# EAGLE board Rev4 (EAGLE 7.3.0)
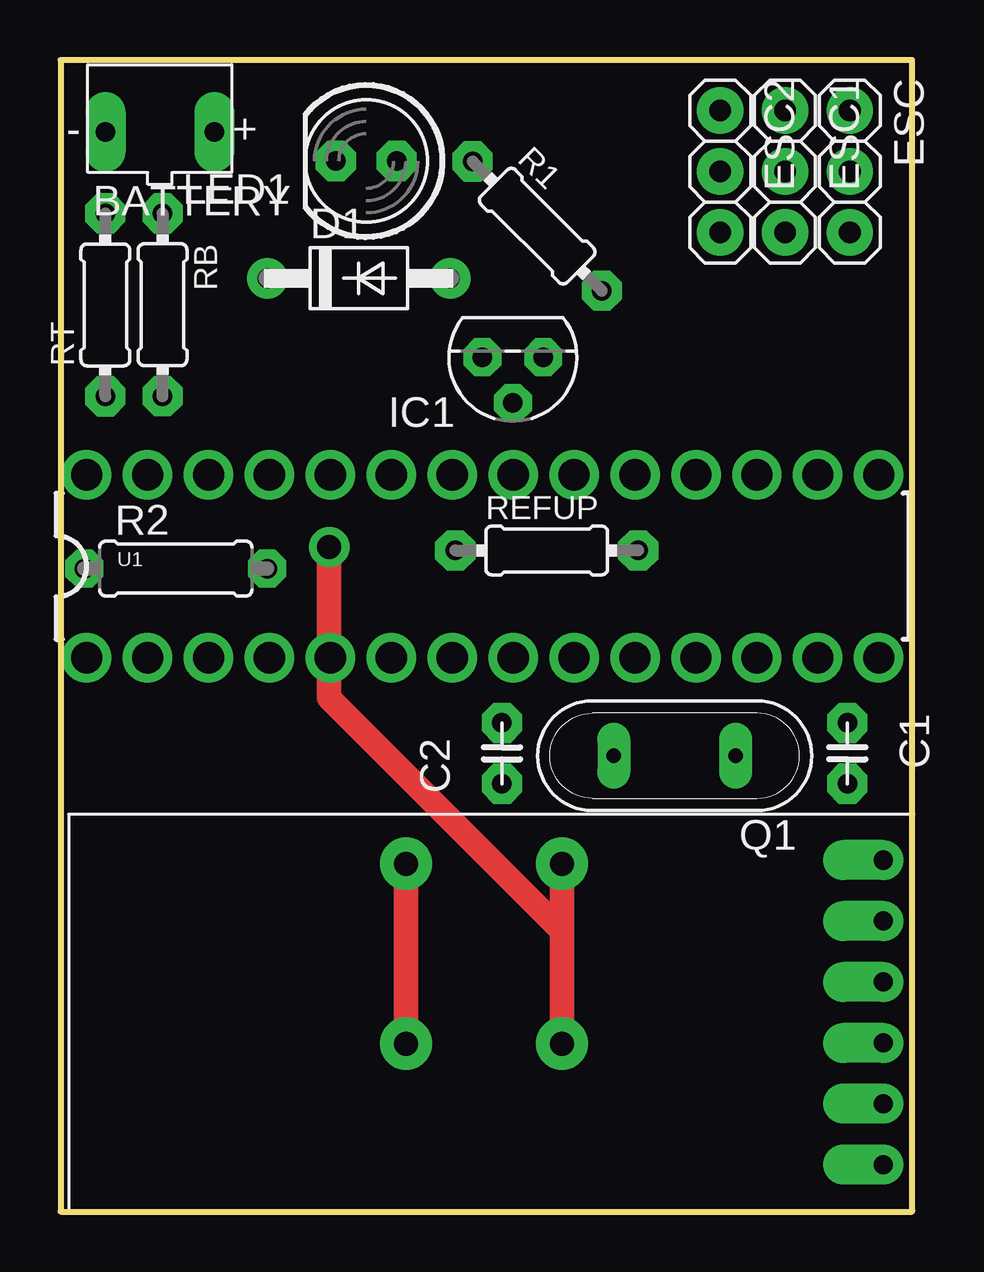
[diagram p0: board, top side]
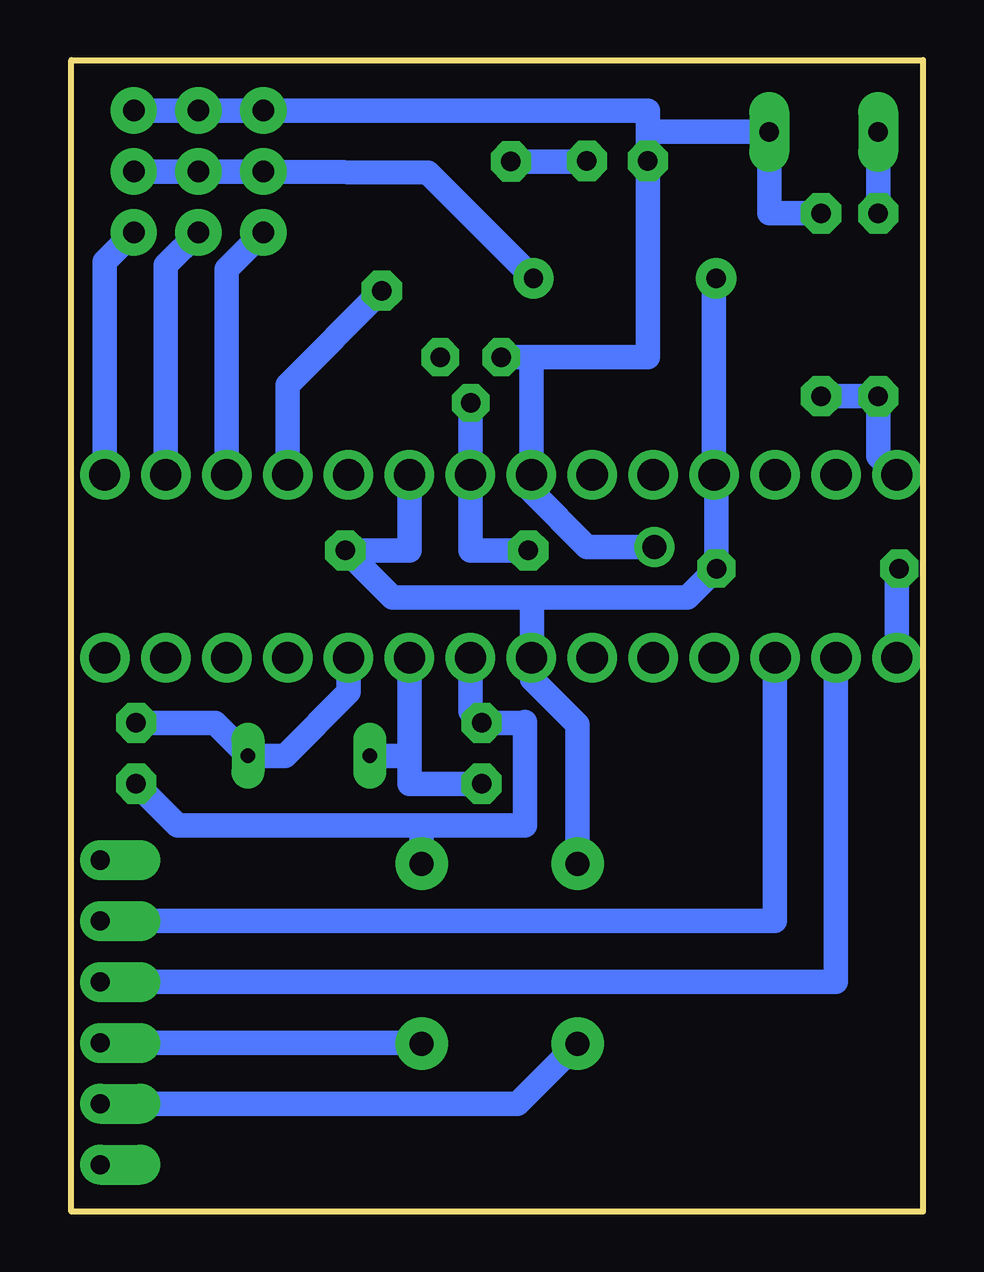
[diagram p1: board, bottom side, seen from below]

Size 35.5 x 48 mm. Coordinates in mm from the lower left corner, seen from the top.
Outline: 0,0 35.5,0 35.5,48 0,48 0,0
Copper layers (1*16): Top 0.035mm / dielectric 1.5mm / Bottom 0.035mm
Design rules "default *": minimum track width 10mil, minimum drill 24mil, track to track 15mil, track to pad 15mil, pad to pad 15mil, via to via 15mil, smd to smd 8mil, copper to edge 15mil, drill to drill 8mil, minimum pad ring 15mil, minimum via ring 8mil, stop-mask expansion 4mil, vias tented up to drill 0mil, thermal gap 10mil

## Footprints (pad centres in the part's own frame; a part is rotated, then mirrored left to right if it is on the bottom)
JST-PH-2-THM = drill 0.8 pad 1.676 long: 1 2.27,0; 2 -2.27,0
C2.5-4 = drill 0.813 pad 1.676 octagon: 1 -1.27,0; 2 1.27,0
DO41-10 = drill 0.8 pad 1.676: A 2.54,0; C -5.08,0
1X03 = drill 0.9 pad 1.93: 1 -2.54,0; 2 0,0; 3 2.54,0
TO92 = drill 0.813 octagon: 1 -1.27,0; 2 0,1.905; 3 1.27,0
LED5MM = drill 0.813 pad 1.676 octagon: A -1.27,0; K 1.27,0
QS = drill 0.61 long: 1 -2.54,0; 2 2.54,0
0204/7 = drill 0.813 pad 1.676 octagon: 1 -3.81,0; 2 3.81,0
0207/7 = drill 0.813 octagon: 1 -3.81,0; 2 3.81,0
DIL28-3 = drill 1.3 pad 1.93: 1 -16.51,-3.81; 2 -13.97,-3.81; 3 -11.43,-3.81; 4 -8.89,-3.81; 5 -6.35,-3.81; 6 -3.81,-3.81; 7 -1.27,-3.81; 8 1.27,-3.81; 9 3.81,-3.81; 10 6.35,-3.81; 11 8.89,-3.81; 12 11.43,-3.81; 13 13.97,-3.81; 14 16.51,-3.81; 15 16.51,3.81; 16 13.97,3.81; 17 11.43,3.81; 18 8.89,3.81; 19 6.35,3.81; 20 3.81,3.81; 21 1.27,3.81; 22 -1.27,3.81; 23 -3.81,3.81; 24 -6.35,3.81; 25 -8.89,3.81; 26 -11.43,3.81; 27 -13.97,3.81; 28 -16.51,3.81
HC06 = drill 0.8 pad 1.676 offset: EN -6.35,0; GND -1.27,0; RX 3.81,0; STATE 6.35,0; TX 1.27,0; VCC -3.81,0

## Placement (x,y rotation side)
BATTERY  [JST-PH-2-THM]  4.14,45 0 top
C1  [C2.5-4]  32.8,19.1 270 top
C2  [C2.5-4]  18.4,19.1 90 top
D1  1N4933  [DO41-10]  13.7,38.9 0 top
ESC  [1X03]  32.9,43.35 270 top
ESC1  [1X03]  30.2,43.35 270 top
ESC2  [1X03]  27.5,43.35 270 top
IC1  LM336LP  [TO92]  18.85,35.61 180 top
LED1  [LED5MM]  12.74,43.79 180 top
Q1  [QS]  25.6,19 180 top
R1  270  [0204/7]  19.87,41.07 315 top
R2  10000  [0207/7]  4.8,26.8 0 top
RB  20000  [0204/7]  4.25,37.8 270 top
REFUP  3300  [0204/7]  20.27,27.55 0 top
RT  220000  [0204/7]  1.86,37.79 90 top
U1  ATMEGA328P_PDIP  [DIL28-3]  17.6,26.89 0 top
U$1  HC06  [HC06]  34.3,8.3 90 top

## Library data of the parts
BATTERY LED1 R1 RB REFUP RT = adafruit
C1 C2 = capacitor-wima
D1 = diode
ESC ESC1 ESC2 = pinhead
IC1 = VLADLIBRARY
Q1 = special
R2 = resistor
U1 = SparkFun-DigitalIC
U$1 = ccs

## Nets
BUTTON: ESC2.3 U1.17
ESC: ESC.3 U1.15
GND: BATTERY.1 C1.2 C2.2 ESC1.1 ESC2.1 ESC.1 IC1.3 LED1.K RB.1 U1.8 U1.22 U$1.GND
LED: R1.2 U1.18
N$2: LED1.A R1.1
N$3: C1.1 Q1.1 U1.10
N$4: BATTERY.2 RT.2
N$5: C2.1 Q1.2 U1.9
N$7: R2.1 U1.1
N$10: D1.A ESC1.2 ESC2.2 ESC.2
RX: U1.2 U$1.TX
STEER: ESC1.3 U1.16
TX: U1.3 U$1.RX
VCC: D1.C R2.2 REFUP.2 U1.7 U1.20 U1.25 U$1.VCC
VOLTMETER: RB.2 RT.1 U1.28
VREF: IC1.2 REFUP.1 U1.21

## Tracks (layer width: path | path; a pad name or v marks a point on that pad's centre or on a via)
BUTTON
  Bottom 1.016: ESC2.3 29.03,39.28 U1.17
ESC
  Bottom 1.016: ESC.3 34.11,39.6 U1.15
GND  (via drill 1 pad 1.68, 1 pad 2.18)
  Top 1.016: v20.9,7 20.9,11.7 | 20.9,11.7 v20.9,14.5 | v11.2,27.7 11.2,21.4 20.9,11.7
  Bottom 1.016: ESC.1 ESC1.1 ESC2.1 11.47,45.89 11.47,45 | U1.8 18.87,20.84 C2.2 16.63,20.37 16.6,20.4 16.6,16.1 20.7,16.1 | C1.2 31.07,16.1 20.7,16.1 | U$1.GND 20.93,7.03 v20.9,7 | v20.9,14.5 20.9,15.9 20.7,16.1 | v11.2,27.7 14,27.7 16.33,30.03 U1.22 16.33,35.61 IC1.3 11.47,35.61 LED1.K 11.47,44.52 11.47,45 | RB.1 6.41,41.61 BATTERY.1 11.47,45
LED
  Bottom 1.016: R1.2 26.49,34.46 U1.18
N$2
  Bottom 1.016: LED1.A 14.01,43.77 R1.1
N$3
  Bottom 1.016: U1.10 23.95,21.65 26.6,19 Q1.1 29.51,20.37 C1.1
N$4
  Bottom 1.016: BATTERY.2 RT.2
N$5
  Bottom 1.016: Q1.2 21.41,19 | 21.41,19 U1.9 | C2.1 21.41,17.83 21.41,19
N$7
  Bottom 1.016: R2.1 1.09,26.7 U1.1
N$10
  Bottom 1.016: D1.A 20.64,43.3 ESC2.2 ESC1.2 ESC.2
RX
  Bottom 1.016: U$1.TX 3.63,9.57 U1.2
STEER
  Bottom 1.016: ESC1.3 31.57,39.44 U1.16
TX
  Bottom 1.016: U$1.RX 6.17,12.11 U1.3
VCC  (via drill 1 pad 2.18)
  Top 1.016: v14.4,7 v14.4,14.5
  Bottom 1.016: U1.20 21.41,27.55 REFUP.2 22.12,25.6 16.3,25.6 | 16.3,25.6 16.3,23.11 U1.7 16.3,23.06 16.3,22.2 14.4,20.3 v14.4,14.5 | 16.3,25.6 9.81,25.6 R2.2 8.61,30.61 U1.25 8.71,38.81 D1.C | U$1.VCC 16.91,4.49 v14.4,7
VOLTMETER
  Bottom 1.016: U1.28 1.86,31.48 RT.1 1.87,33.99 RB.2
VREF
  Bottom 1.016: IC1.2 18.87,33.69 U1.21 18.87,27.55 REFUP.1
